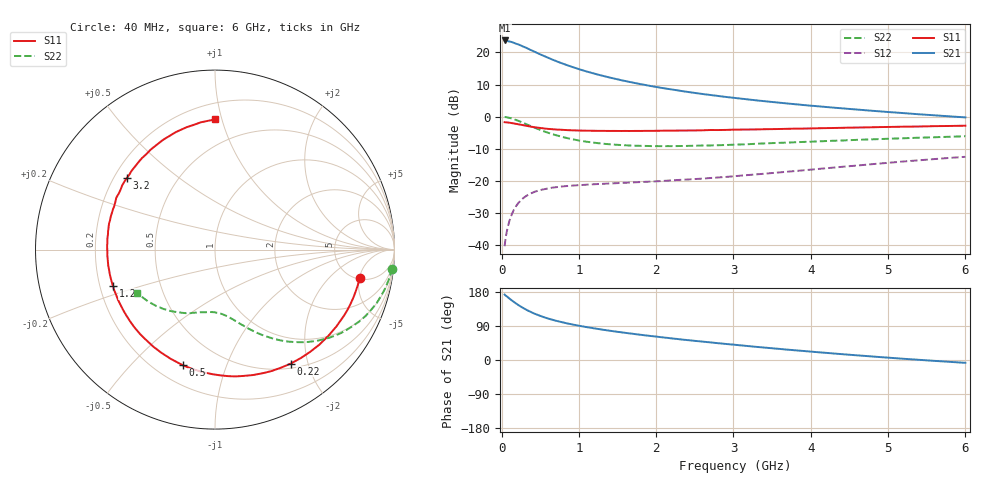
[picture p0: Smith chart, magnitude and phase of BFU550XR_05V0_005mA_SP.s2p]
! Filename:  P:\Prog\Test\Noise\ATS_data\Testdata_Net\03 Spar\BFU550XR_APG2013_45_C05_05p0V_005mA_SP_CM01_D.s2p
! Date/Time: Tue 06/Aug/2013 14:38:16
! BFU550XR_APG2013_45_C05_05p0V_1to35mA_SP_CM01_Bias4_R.s2p
! MDIF S-parameter v. bias file
! BFU550XR_APG2013_45_C05_05p0V_1to35mA_SP_CM01
! Date/time Fri Aug 02 14:46:46 2013
! VAR V_out= 5.0000
! VAR I_out= 5.0000
! VAR V_in= 0.8124
! VAR I_in= 0.0547
! Device data file deembeded for feedlines and parallel
! Original file: \03 Spar\BFU550XR_APG2013_45_C05_05p0V_005mA_SP_CM01_R.s2p
! Feed-files: PR006V01_02082013_Feed1.s2p, PR006V01_02082013_Feed2.s2p
! Parallel-file: PR006V01_02082013_Par.s2p
# MHz S MA R 50
!  Freq-MHz  S11-mag  S11-arg  S21-mag  S21-arg  S12-mag  S12-arg  S22-mag  S22-arg
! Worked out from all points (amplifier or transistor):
!   98 points, 40 MHz to 6 GHz, reference 50 ohm
!   highest |S21| = 23.7 dB at 40 MHz (marker M1)
!   |S21| within 3 dB of that: start of sweep to 380.7 MHz
!   unconditionally stable (mu >= 1): 2.387 GHz to 4.284 GHz
!   at 300 MHz: K = 0.17, MSG = 23.3 dB, |S12| = -25.0 dB
!   at 1.6 GHz: K = 0.78, MSG = 15.8 dB, |S12| = -20.6 dB
!   at 6 GHz: K = 0.85, MSG = 6.1 dB, |S12| = -12.5 dB
!   S11 on the Smith chart (normalised r, x): 40 MHz: 5.27, -5.09; 220 MHz: 0.57, -1.72; 500 MHz: 0.31, -0.71; 1.2 GHz: 0.25, -0.16; 3.2 GHz: 0.25, +0.34; 6 GHz: 0.31, +0.95
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40  0.8225 -10.9  15.4 172.8  0.009661 83.8  0.9901 -6.1
50  0.8201 -13.6  15.37 170.4  0.01206 82.7  0.9882 -7.7
120  0.8006 -32.3  14.7 159.3  0.02764 72.9  0.9488 -18.3
180  0.7783 -47.0  13.84 150.3  0.03917 65.5  0.8982 -26.4
220  0.7625 -56.4  13.33 144.8  0.04566 61.3  0.8608 -31.1
260  0.7466 -64.9  12.68 139.7  0.05136 57.4  0.8234 -35.6
320  0.7216 -77.2  11.83 132.6  0.05846 52.3  0.7662 -41.4
420  0.6884 -94.1  10.38 122.9  0.06718 45.7  0.6813 -49.1
500  0.6689 -105.5  9.366 116.5  0.0722 41.7  0.6246 -54.1
600  0.6474 -117.7  8.307 109.6  0.07647 37.9  0.5638 -59.2
700  0.6327 -127.6  7.402 103.8  0.07982 35.1  0.5175 -63.4
850  0.6192 -139.9  6.335 96.6  0.08354 32.4  0.465 -68.3
1050  0.6085 -152.6  5.285 88.6  0.08672 30.4  0.4171 -73.5
1200  0.604 -160.4  4.692 83.5  0.08893 29.7  0.3938 -76.8
1550  0.6001 -175.2  3.704 73.1  0.09316 29.5  0.362 -83.5
2050  0.605 169.0  2.839 60.5  0.0995 31.4  0.3486 -92.0
2500  0.6112 156.9  2.346 50.5  0.1072 33.7  0.3537 -99.2
3100  0.6314 142.9  1.913 38.5  0.1212 37.1  0.3704 -108.2
3200  0.6325 140.7  1.853 36.6  0.124 37.5  0.3741 -109.6
4100  0.662 122.8  1.452 20.4  0.1541 38.8  0.4133 -123.2
5200  0.6999 103.1  1.139 3.2  0.2011 35.8  0.4625 -139.3
6000  0.7251 90.0  0.9767 -7.5  0.2379 30.9  0.4961 -151.0
